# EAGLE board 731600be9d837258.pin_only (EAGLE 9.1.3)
REV: B

Size 76.2 x 13.97 mm. Coordinates in mm from the lower left corner, seen from the top.
Outline: 0,13.97 0,0 63.01,0 arc22 63.95,0.18 74.6,4.44 arc68 76.2,6.8 76.2,6.92 arc68 74.6,9.28 63.95,13.53 arc22 63.01,13.97 0,13.97
Copper layers (1*16): Top 0.035mm / dielectric 1.5mm / Bottom 0.035mm
Design rules "adafruit *": minimum track width 8mil, minimum drill 15.5mil, track to track 8mil, track to pad 8mil, pad to pad 8mil, via to via 8mil, smd to smd 8mil, copper to edge 10mil, drill to drill 8mil, minimum pad ring 10mil, minimum via ring 8mil, stop-mask expansion 2mil, vias tented up to drill 20mil, thermal gap 10mil
Holes 2.54 mm at 22.86,11.18 22.86,2.54

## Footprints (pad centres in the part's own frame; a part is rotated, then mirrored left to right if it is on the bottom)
0805-NO = smd 1.24 x 1.5: 1 -0.95,0; 2 0.95,0
CHIPLED_0805_NOOUTLINE = smd 1.2 x 1.2: A 0,-1.05; C 0,1.05
FIDUCIAL_1MM = smd 1 x 1: 1 0,0
QFN24_4MM = smd 0.8 x 0.28: 1 -2,1.25; 2 -2,0.75; 3 -2,0.25; 4 -2,-0.25; 5 -2,-0.75; 6 -2,-1.25; 13 2,-1.25; 14 2,-0.75; 15 2,-0.25; 16 2,0.25; 17 2,0.75; 18 2,1.25 | smd 0.28 x 0.8: 7 -1.25,-2; 8 -0.75,-2; 9 -0.25,-2; 10 0.25,-2; 11 0.75,-2; 12 1.25,-2; 19 1.25,2; 20 0.75,2; 21 0.25,2; 22 -0.25,2; 23 -0.75,2; 24 -1.25,2 | smd 1.778 x 1.778: THERM 0,0
SOT363 = smd 0.5 x 0.5: 1 -0.75,-0.9; 3 0.75,-0.9; 4 0.75,0.9; 6 -0.75,0.9 | smd 0.4 x 0.5: 2 0,-0.9; 5 0,0.9
0603-NO = smd 1.075 x 1: 1 -0.85,0; 2 0.85,0
RESPACK_4X0603 = smd 0.45 x 0.9: 1 -1.3,-0.85; 2 -0.4,-0.85; 3 0.4,-0.85; 4 1.3,-0.85; 5 1.3,0.85; 6 0.4,0.85; 7 -0.4,0.85; 8 -1.3,0.85
SOLDERJUMPER_ARROW_NOPASTE = smd 0.762 x 1.524: 1 -1.016,0; 2 1.016,0
TP15R = smd 1.5 x 1.5: TP 0,0
TP10R = smd 1 x 1: TP 0,0
SOT23-5 = smd 0.55 x 1.2: 1 -0.95,-1.3; 2 0,-1.3; 3 0.95,-1.3; 4 0.95,1.3; 5 -0.95,1.3
JSTPH4 = smd 1 x 4.6: 1 -3,-3.7; 2 -1,-3.7; 3 1,-3.7; 4 3,-3.7 | smd 1.7 x 3.4: NC1 -5.7,1.5; NC2 5.7,1.5

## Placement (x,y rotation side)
C3  10uF  [0805-NO]  17.14,3.68 270 top
C5  10uF  [0805-NO]  10.92,4.19 270 top
D1  RED  [CHIPLED_0805_NOOUTLINE]  13.34,1.78 90 top
FID1  FIDUCIAL_1MM  [FIDUCIAL_1MM]  20.07,12.57 0 top
FID2  FIDUCIAL_1MM  [FIDUCIAL_1MM]  2.03,3.81 0 top
IC1  ATSAMD10D14A  [QFN24_4MM]  17.53,9.14 180 top
Q3  2N7002D  [SOT363]  11.68,12.19 90 top
R1  1K  [0603-NO]  18.67,1.91 90 top
R2  1K  [0603-NO]  9.91,1.78 0 top
R6  10K  [RESPACK_4X0603]  11.68,8.76 90 top
SJ8  [SOLDERJUMPER_ARROW_NOPASTE]  5.59,5.59 0 bottom
SJ9  [SOLDERJUMPER_ARROW_NOPASTE]  5.59,8.13 0 bottom
TP1  TPTP15R  [TP15R]  19.81,3.17 0 bottom
TP2  TPTP15R  [TP15R]  19.81,1.02 0 bottom
TP3  TPTP10R  [TP10R]  25.65,6.6 0 top
TP4  TPTP15R  [TP15R]  15.88,5.08 0 bottom
U2  MIC5225-3.3  [SOT23-5]  13.97,4.32 270 top
U$4  [STEMMA_SOIL_BOT]  76.33,0 0 bottom
U$5  [STEMMA_SOIL_TOP]  0,0 0 top
U$12  [PCBFEAT-REV-040]  8.64,5.46 0 bottom
X1  STEMMA_I2C_RASMT  [JSTPH4]  3.56,6.99 90 top

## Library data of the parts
C3 C5 D1 IC1 Q3 R1 R2 R6 U2 U$12 X1 = microbuilder
FID1 FID2 SJ8 SJ9 = microbuilder; BOM: EXCLUDE
TP1-TP4 = testpad
U$4 U$5 = silks

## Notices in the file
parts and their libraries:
microbuilder: This work is placed in the public domain, and may be freely used for commercial and non-commercial work with the following conditions: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
